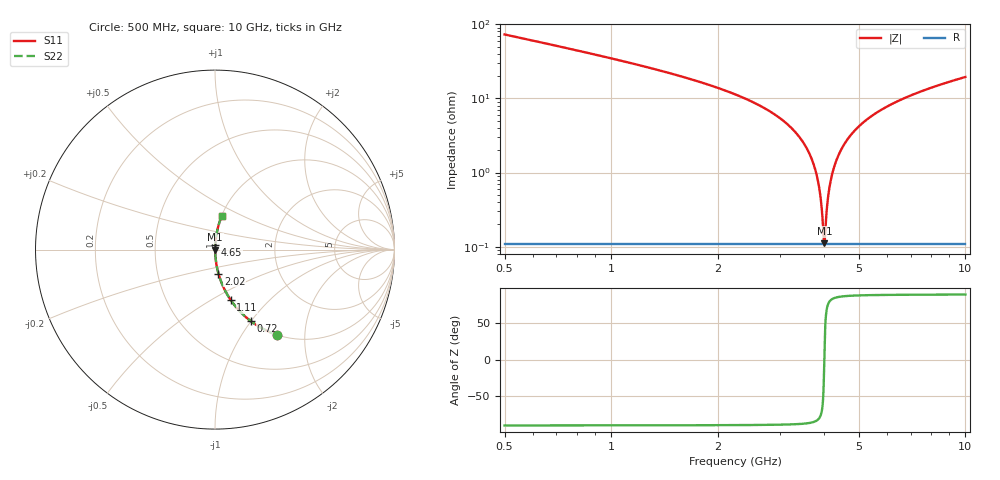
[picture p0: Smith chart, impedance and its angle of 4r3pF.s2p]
! Created Fri Jan 10 15:56:15 2014
# hz S db R 50
! 2 Port Network Data from SP1.SP block
! freq  dbS11  angS11  dbS21  angS21  dbS12  angS12  dbS22  angS22
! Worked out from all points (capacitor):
!   951 points, 500 MHz to 10 GHz, reference 50 ohm
!   read as one part in series: C = 4.3 pF near 540 MHz
!   lowest |Z| = 111 mohm at 4 GHz (marker M1)
!   series resonance near 3.996 GHz, so ESL is about 370 pH
!   S11 on the Smith chart (normalised r, x): 500 MHz: 1.00, -1.46; 720 MHz: 1.00, -0.99; 1.11 GHz: 1.00, -0.62; 2.02 GHz: 1.00, -0.27; 4.65 GHz: 1.00, +0.06; 10 GHz: 1.00, +0.39
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5e8  -4.61 -53.9  -1.86 36.0  -1.86 36.0  -4.61 -53.9
7.2e8  -7.03 -63.5  -0.97 26.4  -0.97 26.4  -7.03 -63.5
1.11e9  -10.64 -72.7  -0.40 17.1  -0.40 17.1  -10.64 -72.7
2.02e9  -17.39 -81.8  -0.09 7.8  -0.09 7.8  -17.39 -81.8
2.09e9  -17.89 -82.2  -0.08 7.3  -0.08 7.3  -17.89 -82.2
3.12e9  -26.70 -86.0  -0.02 2.6  -0.02 2.6  -26.70 -86.0
3.44e9  -31.11 -86.2  -0.01 1.6  -0.01 1.6  -31.11 -86.2
3.67e9  -36.02 -85.1  -0.01 0.9  -0.01 0.9  -36.02 -85.1
3.77e9  -39.30 -83.6  -0.01 0.6  -0.01 0.6  -39.30 -83.6
3.85e9  -43.13 -80.6  -0.01 0.4  -0.01 0.4  -43.13 -80.6
3.91e9  -47.59 -74.6  -0.01 0.2  -0.01 0.2  -47.59 -74.6
3.97e9  -55.77 -48.0  -0.01 0.1  -0.01 0.1  -55.77 -48.0
4e9  -59.14 9.5  -0.01 -0.0  -0.01 -0.0  -59.14 9.5
4.03e9  -54.39 55.1  -0.01 -0.1  -0.01 -0.1  -54.39 55.1
4.11e9  -45.49 77.9  -0.01 -0.3  -0.01 -0.3  -45.49 77.9
4.21e9  -40.25 83.0  -0.01 -0.6  -0.01 -0.6  -40.25 83.0
4.39e9  -35.16 85.4  -0.01 -1.0  -0.01 -1.0  -35.16 85.4
4.65e9  -31.01 86.2  -0.01 -1.6  -0.01 -1.6  -31.01 86.2
5.25e9  -25.84 85.9  -0.02 -2.9  -0.02 -2.9  -25.84 85.9
6.84e9  -19.68 83.4  -0.06 -6.0  -0.06 -6.0  -19.68 83.4
8.42e9  -16.52 81.0  -0.11 -8.6  -0.11 -8.6  -16.52 81.0
1e10  -14.38 78.7  -0.17 -11.0  -0.17 -11.0  -14.38 78.7
